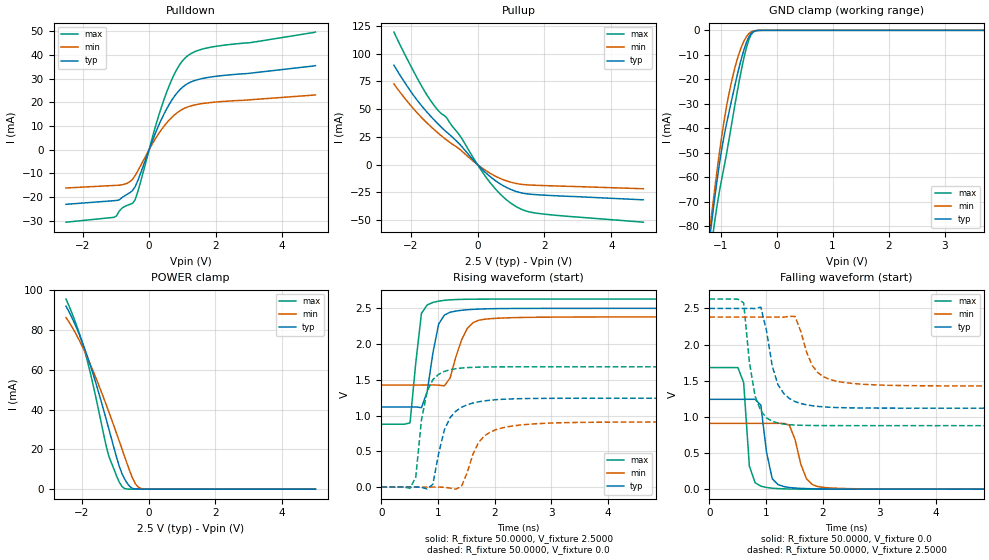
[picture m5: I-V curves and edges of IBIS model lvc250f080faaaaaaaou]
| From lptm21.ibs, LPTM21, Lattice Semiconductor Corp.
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|   Model lvc250f080faaaaaaaou
[Model]   lvc250f080faaaaaaaou
Model_type   Output
Polarity   Non-Inverting
Enable   Active-Low
Vmeas =   1.2500V
Cref =   0.0F
Rref =   1.0000M
Vref =   0.0V
C_comp   4.2000pF   3.8000pF   7.5000pF
[Temperature Range]   25.0000   0.1050k   -40.0000
[Voltage Range]   2.5000V   2.3800V   2.6300V
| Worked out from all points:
|   slope of the pulldown table from 0 to 0.375 V, typ, clamps not added: 28.8 ohm
|   slope of the pullup table from 0 to 0.375 V, typ, clamps not added: 35 ohm
|   GND clamp passes 1 mA (typ) near -0.44 V on its own axis
|   POWER clamp passes 1 mA (typ) near -0.54 V on its own axis
|   rising waveform, R_fixture 50.0000, V_fixture 2.5000: 20-80 % time 177ps typ, 254ps min, 140ps max; typ from 1.12 V to 2.5 V
|   rising waveform, R_fixture 50.0000, V_fixture 0.0: 20-80 % time 281ps typ, 339ps min, 180ps max; typ from 0 V to 1.24 V
|   falling waveform, R_fixture 50.0000, V_fixture 0.0: 20-80 % time 147ps typ, 204ps min, 88.3ps max; typ from 1.24 V to 0 V
|   falling waveform, R_fixture 50.0000, V_fixture 2.5000: 20-80 % time 254ps typ, 299ps min, 194ps max; typ from 2.5 V to 1.12 V
[Pulldown]
|Voltage   I(typ)   I(min)   I(max)
-2.5V     -23.08mA   -16.19mA   -30.63mA
-1.06V    -21.55mA   -15.12mA   -28.59mA
-820mV    -20.29mA   -14.82mA   -24.74mA
-500mV    -17.29mA   -12.49mA   -22.68mA
-420mV    -15.65mA   -10.92mA   -21.14mA
-340mV    -13.01mA   -8.939mA   -17.7mA
220mV     8.066mA    5.348mA    11.25mA
540mV     17.57mA    11.51mA    24.77mA
860mV     24.33mA    15.77mA    34.59mA
1.18V     28.07mA    18.15mA    39.87mA
1.9V      30.77mA    19.97mA    43.38mA
5V        35.47mA    23.12mA    49.65mA
[Pullup]
|Voltage   I(typ)   I(min)   I(max)
-2.5V     89.47mA    72.58mA    119.3mA
-1.96V    64.29mA    51.88mA    86.71mA
-1.4V     43.55mA    34.34mA    57.52mA
-1.16V    35.96mA    27.95mA    48.16mA
-920mV    29.16mA    22.05mA    42.11mA
-520mV    17.92mA    13.48mA    25.76mA
200mV     -6.061mA   -4.41mA    -9.073mA
600mV     -15.83mA   -11.37mA   -24.07mA
920mV     -21.38mA   -15.18mA   -33mA
1.32V     -25.51mA   -17.78mA   -40.3mA
1.72V     -27mA      -18.59mA   -43.55mA
4.96V     -31.72mA   -21.73mA   -51.85mA
[GND_clamp]
|Voltage   I(typ)   I(min)   I(max)
-2.5V     -564.7mA   -543.1mA   -585.2mA
-1.18V    -82.35mA   -79.03mA   -91.15mA
-1.14V    -74.88mA   -71.38mA   -83.96mA
-1.1V     -67.69mA   -63.94mA   -77.25mA
-980mV    -48.66mA   -43.36mA   -60.79mA
-820mV    -30.34mA   -22.65mA   -40.66mA
-700mV    -18.09mA   -11.63mA   -24.79mA
-620mV    -10.87mA   -6.335mA   -15.23mA
-540mV    -5.061mA   -2.654mA   -7.227mA
-460mV    -1.446mA   -714.8uA   -1.98mA
-300mV    -18.71uA   -15.93uA   -16.53uA
5V        0A         0A         0A
[POWER_clamp]
|Voltage   I(typ)   I(min)   I(max)
-2.48V    91.96mA    86.23mA    95.54mA
-2.16V    80.94mA    77.35mA    82.15mA
-1.92V    70.61mA    69.17mA    69.43mA
-1.68V    58.52mA    59.9mA     53.37mA
-1.28V    35.44mA    42.67mA    22.07mA
-1.2V     30.53mA    39.03mA    16.84mA
-960mV    15.8mA     27.82mA    6.447mA
-800mV    7.76mA     20.14mA    1.303mA
-560mV    1.23mA     8.728mA    11.53uA
-400mV    83.98uA    2.726mA    532.6nA
-160mV    776.1nA    102uA      144nA
5V        -44.09nA   -38.33nA   -118.7nA
[Ramp]
| variable   typ   min   max
dV/dt_r  0.7610/0.2778n   0.5462/0.3354n   1.0094/0.1786n
dV/dt_f  0.8277/0.2512n   0.5716/0.2962n   1.0508/0.1921n
R_load = 50.0000
[Rising Waveform]
R_fixture=   50.0000
V_fixture=   2.5000
V_fixture_min=   2.3800
V_fixture_max=   2.6300
|time   V(typ)   V(min)   V(max)
0s        1.121V     1.427V     878.6mV
505.1ps   1.121V     1.427V     897.8mV
606.1ps   1.121V     1.427V     1.734V
707.1ps   1.111V     1.427V     2.431V
808.1ps   1.335V     1.427V     2.547V
1.01ns    2.278V     1.425V     2.601V
1.212ns   2.446V     1.524V     2.619V
1.515ns   2.481V     2.217V     2.627V
1.818ns   2.492V     2.347V     2.629V
10ns      2.5V       2.38V      2.63V
[Rising Waveform]
R_fixture=   50.0000
V_fixture=   0.0
V_fixture_min=   0.0
V_fixture_max=   0.0
|time   V(typ)   V(min)   V(max)
0s        666.9nV    899.8nV    549.6nV
505.1ps   22.6uV     1.285uV    -17.11mV
606.1ps   -46.33uV   988.8nV    136.4mV
707.1ps   -3.152mV   8.393uV    939.9mV
808.1ps   -27.71mV   22.98uV    1.34V
1.212ns   969.8mV    -14.56mV   1.641V
1.414ns   1.115V     9.244mV    1.665V
1.818ns   1.205V     714.8mV    1.679V
2.323ns   1.234V     854.8mV    1.682V
10ns      1.243V     910.3mV    1.682V
[Falling Waveform]
R_fixture=   50.0000
V_fixture=   0.0
V_fixture_min=   0.0
V_fixture_max=   0.0
|time   V(typ)   V(min)   V(max)
0s        1.243V     910.4mV    1.682V
505.1ps   1.243V     910.4mV    1.682V
606.1ps   1.243V     910.4mV    1.473V
707.1ps   1.244V     910.4mV    319.2mV
909.1ps   1.163V     910.3mV    41.68mV
1.01ns    510.6mV    910.3mV    23.4mV
1.212ns   63.63mV    910.5mV    7.931mV
1.717ns   7.747mV    142.5mV    532.8uV
2.02ns    2.628mV    23.7mV     163.4uV
10ns      -16.86uV   10uV       30.14uV
[Falling Waveform]
R_fixture=   50.0000
V_fixture=   2.5000
V_fixture_min=   2.3800
V_fixture_max=   2.6300
|time   V(typ)   V(min)   V(max)
0s        2.5V       2.38V      2.63V
606.1ps   2.5V       2.38V      2.577V
707.1ps   2.501V     2.38V      1.757V
808.1ps   2.498V     2.38V      1.287V
909.1ps   2.519V     2.38V      1.083V
1.212ns   1.445V     2.381V     914.9mV
1.515ns   1.212V     2.389V     887.1mV
1.919ns   1.145V     1.61V      880mV
2.424ns   1.126V     1.472V     878.8mV
10ns      1.121V     1.427V     878.6mV
